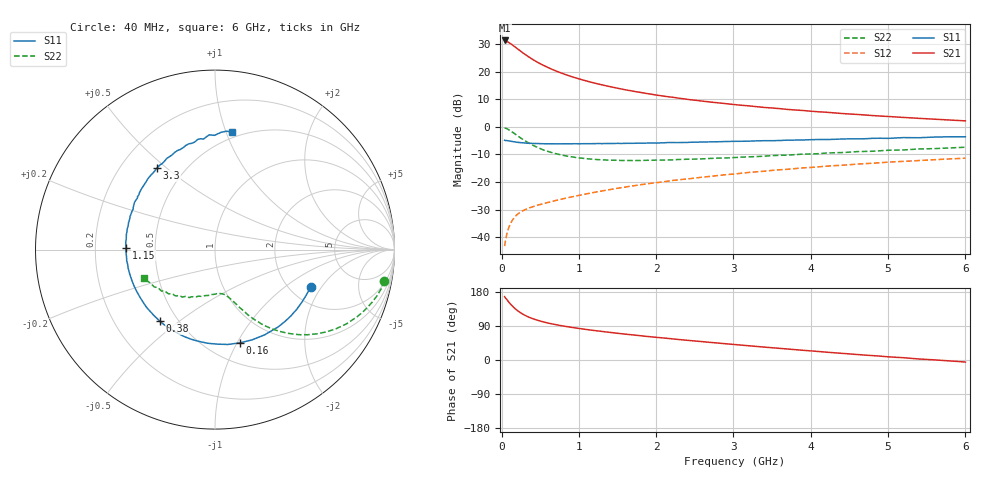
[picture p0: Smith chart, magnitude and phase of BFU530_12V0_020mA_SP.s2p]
! Filename:  P:\Prog\Test\Noise\ATS_data\Testdata_Net\03 Spar\BFU530_APG2013_40_A05_12p0V_020mA_SP_CM01_D.s2p
! Date/Time: Fri 26/Apr/2013 13:03:12
! BFU530_APG2013_40_A05_12p0V_1to25mA_SP_CM01_Bias7_R.s2p
! MDIF S-parameter v. bias file
! BFU530_APG2013_40_A05_12p0V_1to25mA_SP_CM01
! Date/time Wed Apr 24 20:41:12 2013
! VAR V_out= 12.0010
! VAR I_out= 19.9950
! VAR V_in= 0.7882
! VAR I_in= 0.1952
! Device data file deembeded for feedlines and parallel
! Original file: \03 Spar\BFU530_APG2013_40_A05_12p0V_020mA_SP_CM01_R.s2p
! Feed-files: PR047V01_250413_Feed1.s2p, PR047V01_250413_Feed2.s2p
! Parallel-file: PR047V01_250413_Par.s2p
# MHz S MA R 50
!  Freq-MHz  S11-mag  S11-arg  S21-mag  S21-arg  S12-mag  S12-arg  S22-mag  S22-arg
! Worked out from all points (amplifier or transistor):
!   98 points, 40 MHz to 6 GHz, reference 50 ohm
!   highest |S21| = 31.4 dB at 40 MHz (marker M1)
!   |S21| within 3 dB of that: start of sweep to 205.2 MHz
!   unconditionally stable (mu >= 1): 1.439 GHz to 3.767 GHz
!   at 300 MHz: K = 0.45, MSG = 28.3 dB, |S12| = -30.1 dB
!   at 1.6 GHz: K = 1.02, MAG = 16.8 dB, |S12| = -21.8 dB
!   at 6 GHz: K = 0.88, MSG = 6.8 dB, |S12| = -11.3 dB
!   S11 on the Smith chart (normalised r, x): 40 MHz: 2.59, -1.59; 160 MHz: 0.70, -1.02; 380 MHz: 0.40, -0.43; 1.15 GHz: 0.34, +0.01; 3.3 GHz: 0.35, +0.47; 6 GHz: 0.45, +1.05
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40  0.5726 -21.1  37.03 167.4  0.006859 79.5  0.9593 -10.4
50  0.5684 -26.5  36.83 163.9  0.008507 77.8  0.9516 -13.2
100  0.5563 -50.7  33.52 151.5  0.01568 69.7  0.8764 -25.2
120  0.5497 -59.7  32.23 146.6  0.0181 66.7  0.8417 -29.4
160  0.5375 -75.3  29.28 138.4  0.02222 61.7  0.7704 -36.6
200  0.527 -88.6  26.54 131.4  0.02549 58.0  0.7016 -42.5
260  0.5169 -105.0  22.96 122.8  0.02923 54.5  0.6135 -49.3
320  0.5084 -117.6  19.99 116.2  0.03222 52.4  0.543 -54.4
380  0.5033 -127.7  17.56 110.9  0.03468 51.2  0.4859 -58.1
440  0.4994 -135.8  15.62 106.5  0.03697 50.9  0.4408 -61.0
500  0.4972 -142.6  14.03 102.9  0.03913 50.9  0.4053 -63.4
650  0.4945 -155.8  11.14 95.4  0.04438 51.9  0.3427 -67.7
850  0.4946 -167.8  8.694 88.0  0.05157 53.6  0.2946 -71.6
1050  0.4957 -177.5  7.114 81.8  0.05909 55.0  0.2698 -75.3
1150  0.4966 178.7  6.516 79.1  0.06297 55.5  0.261 -76.8
1600  0.503 163.8  4.722 68.2  0.08097 56.4  0.2464 -84.5
2050  0.5129 152.7  3.696 58.9  0.09917 55.8  0.2498 -92.6
3100  0.5486 129.1  2.474 39.3  0.1442 51.5  0.2827 -111.5
3300  0.5583 125.2  2.329 35.8  0.1533 50.3  0.2894 -114.9
4100  0.5903 110.6  1.881 22.4  0.1885 44.7  0.327 -128.5
5200  0.6403 92.9  1.486 6.0  0.2373 35.9  0.3822 -146.2
6000  0.6626 81.8  1.288 -5.4  0.2708 28.6  0.428 -158.4
